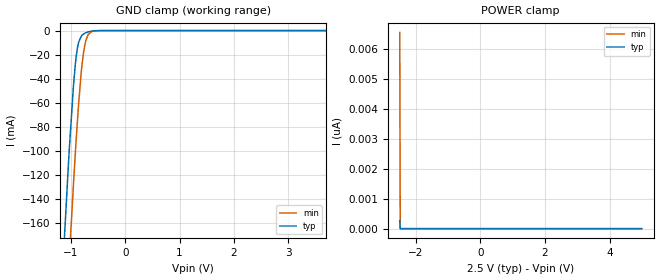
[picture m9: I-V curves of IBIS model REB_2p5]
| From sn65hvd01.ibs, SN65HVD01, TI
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|   Model
[Model]   REB_2p5
Model_type   Input
Vinl = 0.75
Vinh = 1.75
|   typ   min   max
C_comp   1pF   1pF   1pF
[Voltage Range]   2.5   2.25   NA
[Temperature Range]   27   125   NA
[Power Clamp Reference]   2.5   2.25   NA
[GND Clamp Reference]   -0   -0   NA
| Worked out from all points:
|   GND clamp passes 1 mA (typ) near -0.68 V on its own axis
[GND Clamp]
|   Voltage   I(typ)   I(min)   I(max)
-2.5V     -1.489A    -1.579A    NA
-1.135V   -184mA     -278.8mA   NA
-1.03V    -97.77mA   -188.5mA   NA
-955mV    -46.16mA   -128.1mA   NA
-902.5mV  -20.92mA   -89.34mA   NA
-857.5mV  -9.447mA   -59.73mA   NA
-812.5mV  -4.773mA   -35.19mA   NA
-767.5mV  -2.795mA   -17.56mA   NA
-730mV    -1.837mA   -8.672mA   NA
-625mV    -447uA     -991.3uA   NA
-497.5mV  -41.76uA   -87.9uA    NA
4.992V    0A         0A         NA
[POWER Clamp]
|   Voltage   I(typ)   I(min)   I(max)
-2.5V     271.1pA    6.559nA    NA
-2.485V   0A         0A         NA
-2.478V   0A         0A         NA
4.992V    0A         0A         NA
